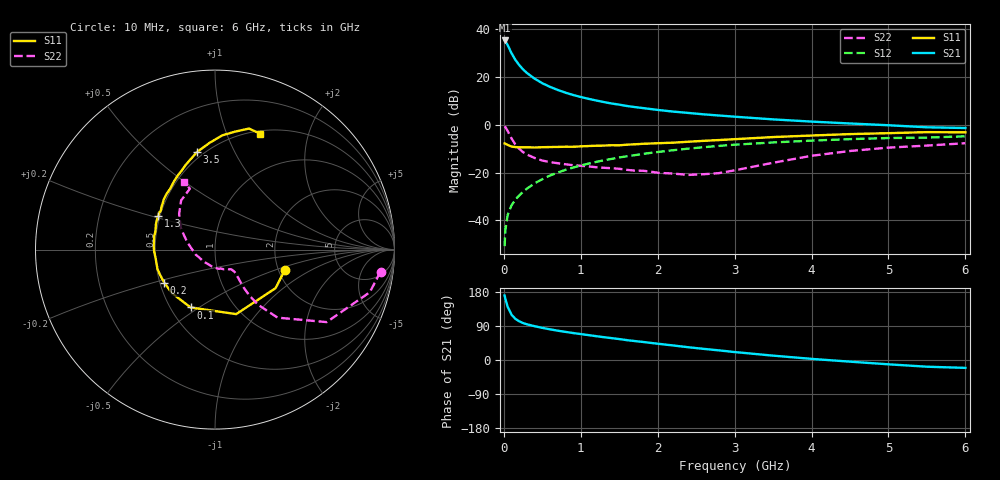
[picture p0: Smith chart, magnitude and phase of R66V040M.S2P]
! SIEMENS Small Signal Semiconductors
! BFR193
! Si NPN RF Bipolar Junction Transistor in SOT23
! VCE = 6 V  IC = 40 mA
! Common Emitter S-Parameters:  May  1996
# GHz  S  MA  R  50
!  f  S11  S21  S12  S22
! GHz  MAG  ANG  MAG  ANG  MAG  ANG  MAG  ANG
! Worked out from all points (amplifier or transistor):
!   36 points, 10 MHz to 6 GHz, reference 50 ohm
!   highest |S21| = 35.2 dB at 10 MHz (marker M1)
!   |S21| within 3 dB of that: start of sweep to 65.27 MHz
!   unconditionally stable (mu >= 1): 445.1 MHz to 2.032 GHz
!   at 250 MHz: K = 0.92, MSG = 25.6 dB, |S12| = -28.0 dB
!   at 1.4 GHz: K = 1.02, MAG = 10.7 dB, |S12| = -14.3 dB
!   at 6 GHz: K = 0.95, MSG = 1.7 dB, |S12| = -4.8 dB
!   S11 on the Smith chart (normalised r, x): 10 MHz: 2.16, -0.59; 100 MHz: 0.63, -0.46; 200 MHz: 0.53, -0.22; 1.3 GHz: 0.49, +0.21; 3.5 GHz: 0.46, +0.72; 6 GHz: 0.53, +1.32
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0.01  0.4054 -16.4  57.71 170.2  0.0029 85.9  0.9305 -7.6
0.02  0.4 -32.5  55.75 161.2  0.0064 78.3  0.8945 -15.4
0.05  0.3784 -71.8  45.96 140.1  0.013 70.8  0.7418 -33.0
0.1  0.3499 -112.8  31.26 119.6  0.0207 67.0  0.5151 -47.4
0.15  0.3412 -134.4  22.66 108.6  0.0273 67.8  0.3878 -52.1
0.2  0.3378 -146.8  17.64 102.1  0.0332 69.2  0.3149 -53.2
0.25  0.3371 -155.8  14.31 97.5  0.0397 70.8  0.2673 -52.9
0.3  0.3382 -161.3  12.06 94.2  0.0462 72.0  0.2386 -52.2
0.4  0.3344 -171.7  9.186 89.2  0.0596 72.5  0.2022 -50.5
0.5  0.3391 -178.3  7.373 84.8  0.0728 72.9  0.1783 -49.1
0.6  0.342 176.8  6.192 81.0  0.0868 72.6  0.1658 -48.8
0.7  0.3437 172.0  5.34 77.4  0.1003 71.7  0.1571 -49.2
0.8  0.3469 167.7  4.688 74.3  0.1138 70.6  0.1493 -49.8
0.9  0.3467 163.7  4.189 71.2  0.1272 69.8  0.1427 -50.3
1.1  0.3588 156.5  3.483 65.7  0.154 67.5  0.1346 -54.8
1.3  0.3668 149.3  2.979 60.2  0.1808 64.8  0.1259 -59.3
1.7  0.3897 138.3  2.341 50.0  0.2313 59.2  0.1099 -73.5
2.2  0.4218 126.2  1.883 38.4  0.2935 52.0  0.0954 -101.2
3.5  0.5527 100.5  1.294 11.5  0.4267 31.8  0.1605 164.9
4.5  0.6375 86.4  1.062 -4.4  0.5002 17.8  0.2828 135.0
5.5  0.7005 74.3  0.884 -17.7  0.5388 4.1  0.367 112.4
6  0.6933 68.8  0.854 -20.8  0.5732 0.2  0.4113 114.6
